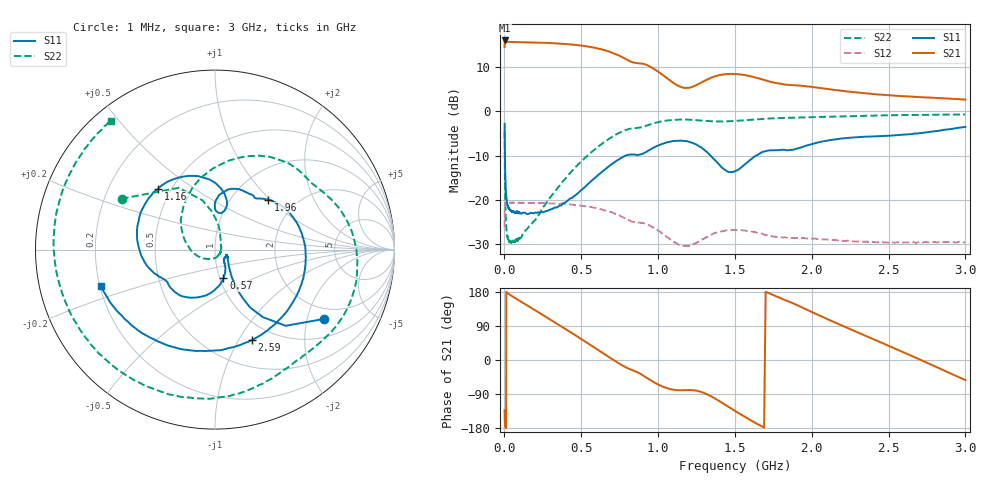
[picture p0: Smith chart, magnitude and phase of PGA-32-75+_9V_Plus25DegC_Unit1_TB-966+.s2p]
!Mini-Circuits Laboratory
!S-Parameters
!Model: PGA-32-75+
!Run / Lot / Date Code: Q18610 / CP621-001-03-01EV / 1724
!Fixture: TB-966+_ED17052601
!Network Analyzer: PNA-X N5244A - 423 4 ports;  Serial number: 74314
!Date: 7/21/2017 at 2:35:23 PM
!S/N: Unit# 1
!Tested with:
# Hz  S  dB  R  50
!Frequency  S11 dB  S11 Deg  S21 dB  S21 Deg  S12 dB  S12 Deg  S22 dB  S22 Deg
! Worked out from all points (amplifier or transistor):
!   399 points, 1 MHz to 3 GHz, reference 50 ohm
!   highest |S21| = 16.0 dB at 2.5 MHz (marker M1)
!   |S21| within 3 dB of that: start of sweep to 719.2 MHz
!   unconditionally stable (mu >= 1): start of sweep to end of sweep
!   at 58 MHz: K = 1.17, MAG = 15.7 dB, |S12| = -20.6 dB
!   at 1.01 GHz: K = 1.59, MAG = 13.4 dB, |S12| = -27.1 dB
!   at 3 GHz: K = 1.48, MAG = 12.0 dB, |S12| = -29.5 dB
!   S11 on the Smith chart (normalised r, x): 1 MHz: 1.59, -2.56; 570 MHz: 1.04, -0.34; 1.16 GHz: 0.42, +0.37; 1.96 GHz: 1.46, +0.98; 2.59 GHz: 0.80, -1.14; 3 GHz: 0.20, -0.15
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1000000  -2.84 -32.3  14.51 -132.4  -26.18 89.1  -4.54 151.5
1500000  -4.75 -47.2  15.82 -150.4  -22.62 63.6  -7.97 120.5
2500000  -8.47 -58.7  16.01 -165.0  -21.31 37.4  -13.32 95.1
8000000  -17.21 -53.5  15.71 -177.9  -20.72 10.2  -23.70 60.8
3.8e7  -22.31 -27.1  15.68 171.4  -20.65 -5.2  -29.54 -2.0
1.4e8  -23.04 -35.2  15.60 145.9  -20.65 -27.9  -26.77 -86.3
2.4e8  -22.67 -46.0  15.50 121.3  -20.74 -49.0  -22.33 -139.2
3.8e8  -20.74 -54.8  15.26 86.3  -20.91 -78.6  -15.78 168.4
5.1e8  -17.50 -64.5  14.80 52.9  -21.35 -107.5  -11.04 130.3
5.7e8  -15.58 -73.6  14.47 37.0  -21.64 -120.9  -9.12 113.2
6.7e8  -12.66 -92.7  13.62 10.4  -22.48 -143.7  -6.47 86.3
7.7e8  -10.31 -119.0  12.18 -15.0  -23.90 -165.1  -4.46 59.9
1.01e9  -7.59 -178.2  8.73 -66.5  -27.15 152.8  -2.37 9.6
1.16e9  -6.64 133.1  5.37 -79.8  -30.35 145.5  -1.85 -19.4
1.31e9  -8.98 87.0  7.04 -88.8  -28.48 141.9  -2.16 -42.3
1.51e9  -13.38 88.0  8.41 -136.8  -26.82 101.5  -2.14 -65.1
1.65e9  -9.73 81.1  7.50 -169.8  -27.47 73.3  -1.79 -81.8
1.96e9  -7.80 43.1  5.68 134.2  -28.71 27.5  -1.35 -122.1
2.01e9  -7.32 37.0  5.47 124.9  -28.78 19.9  -1.30 -128.2
2.51e9  -5.47 -50.3  3.62 35.8  -29.49 -54.9  -0.89 173.0
2.59e9  -5.30 -67.9  3.42 21.6  -29.64 -67.0  -0.85 164.9
3e9  -3.51 -162.4  2.65 -53.0  -29.55 -131.6  -0.70 128.9
